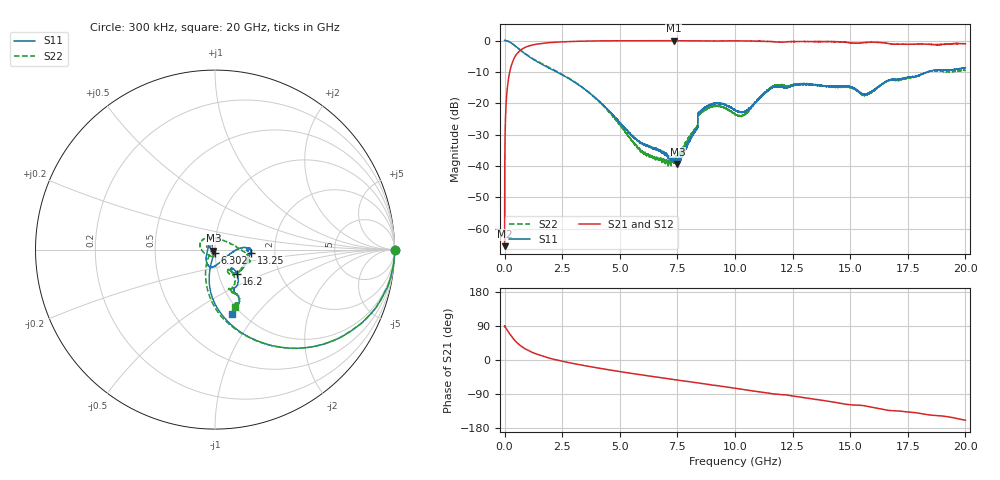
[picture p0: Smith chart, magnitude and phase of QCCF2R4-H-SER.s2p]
!QCCF2R4
!Johanson Technology Inc.
!www.johansontechnology.com
!Test Board Conditions:
!Substrate Type  RO4350B
!Substrate Thickness  10 mil
!Substrate Dk  3.66
!TL Type: GCPW
!TL Trace Width  21 mil
!TL Gap  20 mil
!Electrode orientation  Horizontal
!DUT TOPOLOGY	SERIES
!Mounting Pad LxW  16x21 mil
# MHz S  dB  R 50
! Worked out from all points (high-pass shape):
!   20001 points, 300 kHz to 20 GHz, reference 50 ohm
!   highest |S21| = -0.03 dB at 7.332 GHz (marker M1); lowest = -65.5 dB at 300 kHz (marker M2)
!   |S21| within 3 dB of the highest: 698.6 MHz to end of sweep
!   lowest |S11| = -39.3 dB at 7.501 GHz (marker M3), VSWR 1.02, Z = 49.2 - j0.656 ohm
!   |S11| at or under -10 dB: 2.263 GHz to 18.33 GHz (16.07 GHz wide, 156 % of centre); 18.33243 GHz to 18.33383 GHz (1.4 MHz wide, 0.00764 % of centre); 18.33527 GHz to 18.33634 GHz (1.066 MHz wide, 0.00581 % of centre)
!   |S22| runs from -39.9 to 0.0 dB; largest |S21 - S12| = 0.028
!   S11 on the Smith chart (normalised r, x): 300 kHz: open; 6.302 GHz: 1.00, -0.04; 13.25 GHz: 1.50, -0.05; 16.2 GHz: 1.23, -0.34; 20 GHz: 0.92, -0.76
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0.3  0.03 -0.1  -65.51 88.5  -66.75 95.0  0.03 -0.0
101.298  -0.10 -9.7  -16.41 80.1  -16.42 80.2  -0.09 -9.7
125.298  -0.14 -12.0  -14.62 77.7  -14.63 77.9  -0.15 -12.1
243.296  -0.55 -22.5  -9.30 67.0  -9.30 67.2  -0.57 -22.6
439.293  -1.59 -37.4  -5.30 51.9  -5.29 52.1  -1.60 -37.5
1375.279  -6.56 -73.9  -1.17 15.9  -1.15 15.7  -6.41 -73.5
3334.25  -14.73 -100.0  -0.21 -13.3  -0.20 -13.3  -14.68 -105.7
6302.205  -33.81 -89.0  -0.07 -42.4  -0.07 -42.4  -36.90 -172.2
6667.2  -34.95 -90.6  -0.06 -45.7  -0.07 -45.6  -37.91 -174.5
7332.19  -38.33 -121.2  -0.03 -51.4  -0.05 -51.4  -38.21 -147.3
7501.187  -39.32 -141.9  -0.08 -52.9  -0.07 -53.0  -37.37 -134.6
8286.176  -28.83 151.7  -0.08 -59.6  -0.07 -59.6  -28.11 -101.2
8603.171  -21.89 -126.4  -0.10 -62.5  -0.11 -62.5  -22.61 -177.8
10000.15  -22.11 -73.4  -0.09 -74.6  -0.11 -74.4  -23.48 103.1
10488.14  -22.38 -31.2  -0.14 -79.1  -0.09 -78.9  -23.19 46.8
11690.12  -14.64 1.2  -0.42 -89.6  -0.39 -90.0  -14.39 -12.5
13251.1  -13.91 -4.7  -0.31 -101.6  -0.28 -101.5  -13.81 -20.2
13334.1  -14.09 -5.8  -0.33 -102.3  -0.35 -102.4  -14.01 -21.2
15597.07  -17.13 -50.8  -0.66 -120.5  -0.61 -121.0  -17.30 -58.1
16196.06  -14.82 -47.8  -0.56 -127.8  -0.48 -128.2  -14.92 -53.7
16667.05  -12.64 -58.0  -0.94 -132.9  -0.92 -133.7  -12.64 -63.9
20000  -8.66 -74.7  -1.02 -158.9  -0.86 -157.8  -9.38 -71.1
